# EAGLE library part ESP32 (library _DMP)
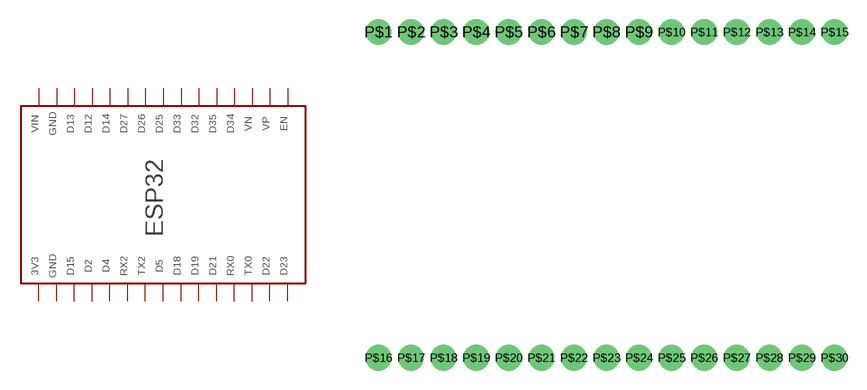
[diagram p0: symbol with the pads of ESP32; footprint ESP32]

Designator prefix -

## ESP32  [ESP32]
P$1  VIN
P$2  GND
P$3  D13
P$4  D12
P$5  D14
P$6  D27
P$7  D26
P$8  D25
P$9  D33
P$10  D32
P$11  D35
P$12  D34
P$13  VN
P$14  VP
P$15  EN
P$16  3V3
P$17  GND2
P$18  D15
P$19  D2
P$20  D4
P$21  RX2
P$22  TX2
P$23  D5
P$24  D18
P$25  D19
P$26  D21
P$27  RX0
P$28  TX0
P$29  D22
P$30  D23

## Footprint ESP32 (pad centres in mm)
drill 1.1 pad 2: P$1 0,0; P$2 2.54,0; P$3 5.08,0; P$4 7.62,0; P$5 10.16,0; P$6 12.7,0; P$7 15.24,0; P$8 17.78,0; P$9 20.32,0; P$10 22.86,0; P$11 25.4,0; P$12 27.94,0; P$13 30.48,0; P$14 33.02,0; P$15 35.56,0; P$16 0,-25.4; P$17 2.54,-25.4; P$18 5.08,-25.4; P$19 7.62,-25.4; P$20 10.16,-25.4; P$21 12.7,-25.4; P$22 15.24,-25.4; P$23 17.78,-25.4; P$24 20.32,-25.4; P$25 22.86,-25.4; P$26 25.4,-25.4; P$27 27.94,-25.4; P$28 30.48,-25.4; P$29 33.02,-25.4; P$30 35.56,-25.4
